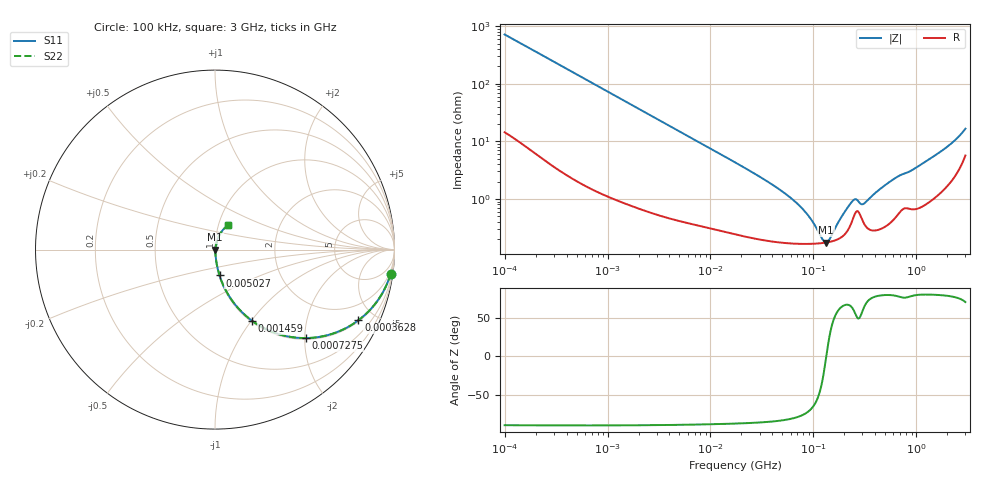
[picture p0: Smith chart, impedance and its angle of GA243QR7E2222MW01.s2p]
!Murata Part Number: GA243QR7E2222MW01
!These Parameters are Measured in Series Mode Connection
!Data Generated on Jun 19, 2026
!  o--ll--o
!Port1  Port2
!  o------o
!Operation Temp=25[degC], DC Bias Voltage=0[V]
!Freq. Start=100[kHz] Stop=3[GHz] 401[Steps]
# Hz S RI R 50
!Freq.(Hz) S11(Real) S11(Imag) S21(Real) S21(Imag) S12(Real) S12(Imag) S22(Real) S22(Imag)
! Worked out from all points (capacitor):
!   401 points, 100 kHz to 3 GHz, reference 50 ohm
!   read as one part in series: C = 2.2 nF near 105.3 kHz
!   lowest |Z| = 174 mohm at 132.7 MHz (marker M1)
!   series resonance near 133.5 MHz, so ESL is about 650 pH
!   S11 on the Smith chart (normalised r, x): 100 kHz: 1, -14; 362.8 kHz: 1.06, -4.03; 727.5 kHz: 1.03, -2.02; 1.459 MHz: 1.02, -1.01; 5.027 MHz: 1.01, -0.30; 3 GHz: 1.11, +0.31
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100000  0.9785 -0.1355  0.0215 0.1355  0.0215 0.1355  0.9785 -0.1355
205778  0.9222 -0.2597  0.0778 0.2597  0.0778 0.2597  0.9222 -0.2597
362777  0.7988 -0.3938  0.2012 0.3938  0.2012 0.3938  0.7988 -0.3938
562235  0.6277 -0.4765  0.3723 0.4765  0.3723 0.4765  0.6277 -0.4765
727522  0.5042 -0.493  0.4958 0.493  0.4958 0.493  0.5042 -0.493
1458987  0.2073 -0.3972  0.7927 0.3972  0.7927 0.3972  0.2073 -0.3972
3161081  0.0565 -0.2202  0.9435 0.2202  0.9435 0.2202  0.0565 -0.2202
5026967  0.0253 -0.1437  0.9747 0.1437  0.9747 0.1437  0.0253 -0.1437
1.77727e7  0.00414 -0.0417  0.9959 0.0417  0.9959 0.0417  0.00414 -0.0417
5.523785e7  0.00183 -0.0116  0.9982 0.0116  0.9982 0.0116  0.00183 -0.0116
7.722238e7  0.00169 -0.0067  0.9983 0.0067  0.9983 0.0067  0.00169 -0.0067
9.738194e7  0.00167 -0.00377  0.9983 0.00377  0.9983 0.00377  0.00167 -0.00377
1.228043e8  0.0017 -0.000995  0.9983 0.000995  0.9983 0.000995  0.0017 -0.000995
1.326759e8  0.00174 -7.64e-05  0.9983 7.64e-05  0.9983 7.64e-05  0.00174 -7.64e-05
1.43341e8  0.00178 0.000854  0.9982 -0.000854  0.9982 -0.000854  0.00178 0.000854
1.854806e8  0.00214 0.00419  0.9979 -0.00419  0.9979 -0.00419  0.00214 0.00419
2.400085e8  0.00433 0.00802  0.9957 -0.00802  0.9957 -0.00802  0.00433 0.00802
2.593015e8  0.00596 0.00779  0.994 -0.00779  0.994 -0.00779  0.00596 0.00779
3.105665e8  0.00376 0.00735  0.9962 -0.00735  0.9962 -0.00735  0.00376 0.00735
5.475153e8  0.00405 0.0191  0.9959 -0.0191  0.9959 -0.0191  0.00405 0.0191
1.616196e9  0.0148 0.0586  0.9852 -0.0586  0.9852 -0.0586  0.0148 0.0586
3e9  0.0737 0.1365  0.9263 -0.1365  0.9263 -0.1365  0.0737 0.1365
